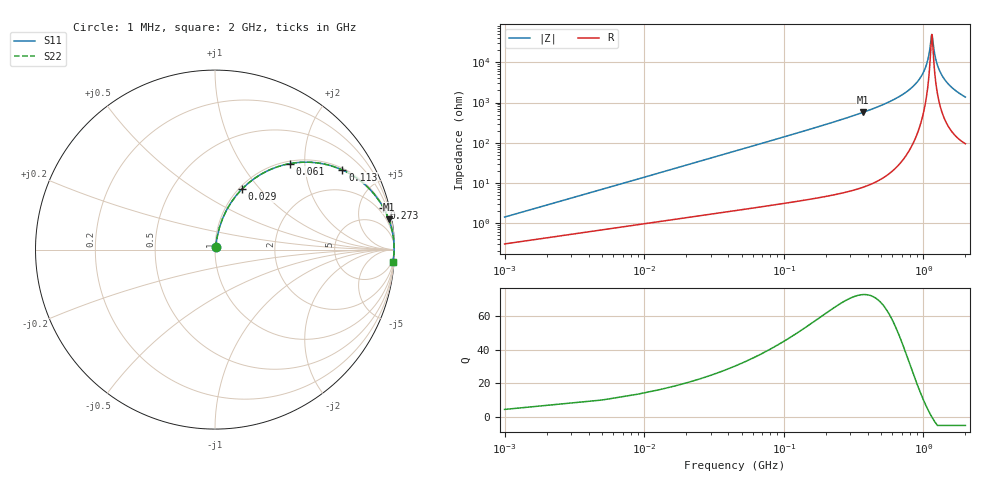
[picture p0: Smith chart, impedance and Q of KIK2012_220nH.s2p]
!version-2
!date-01.2022
!Series
# MHz S RI R 50
!Freq ReS11 ImS11 ReS21 ImS21 ReS12 ImS12 ReS22 ImS22
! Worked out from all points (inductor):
!   501 points, 1 MHz to 2 GHz, reference 50 ohm
!   read as one part in series: L = 220 nH near 9 MHz
!   highest Q = 72.9 at 369 MHz (marker M1), where L = 245 nH
!   self-resonance near 1.149 GHz
!   S11 on the Smith chart (normalised r, x): 1 MHz: 1.01, +0.03; 29 MHz: 1.03, +0.80; 61 MHz: 1.05, +1.69; 113 MHz: 1.07, +3.15; 273 MHz: 1.12, +8.00; 2 GHz: 3, -27
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1  0.00322 0.0137  0.9968 -0.0137  0.9968 -0.0137  0.00322 0.0137
13  0.0411 0.1705  0.9589 -0.1705  0.9589 -0.1705  0.0411 0.1705
21  0.0885 0.261  0.9115 -0.261  0.9115 -0.261  0.0885 0.261
29  0.1487 0.336  0.8513 -0.336  0.8513 -0.336  0.1487 0.336
61  0.4193 0.4795  0.5807 -0.4795  0.5807 -0.4795  0.4193 0.4795
113  0.7094 0.4437  0.2906 -0.4437  0.2906 -0.4437  0.7094 0.4437
177  0.8585 0.3402  0.1415 -0.3402  0.1415 -0.3402  0.8585 0.3402
273  0.9382 0.2337  0.0618 -0.2337  0.0618 -0.2337  0.9382 0.2337
337  0.9605 0.188  0.0395 -0.188  0.0395 -0.188  0.9605 0.188
369  0.9678 0.1698  0.0322 -0.1698  0.0322 -0.1698  0.9678 0.1698
669  0.9935 0.071  0.00654 -0.071  0.00654 -0.071  0.9935 0.071
869  0.9972 0.0356  0.00281 -0.0356  0.00281 -0.0356  0.9972 0.0356
1001  0.998 0.0175  0.00203 -0.0175  0.00203 -0.0175  0.998 0.0175
1081  0.9981 0.00784  0.00193 -0.00784  0.00193 -0.00784  0.9981 0.00784
1149  0.998 0.000199  0.00201 -0.000199  0.00201 -0.000199  0.998 0.000199
1161  0.998 -0.0011  0.00204 0.0011  0.00204 0.0011  0.998 -0.0011
1193  0.9979 -0.0045  0.00213 0.0045  0.00213 0.0045  0.9979 -0.0045
1229  0.9977 -0.00822  0.00227 0.00822  0.00227 0.00822  0.9977 -0.00822
1337  0.9972 -0.0188  0.00285 0.0188  0.00285 0.0188  0.9972 -0.0188
1473  0.9961 -0.0311  0.00388 0.0311  0.00388 0.0311  0.9961 -0.0311
1669  0.9941 -0.0473  0.00586 0.0473  0.00586 0.0473  0.9941 -0.0473
2000  0.9898 -0.0718  0.0102 0.0718  0.0102 0.0718  0.9898 -0.0718
